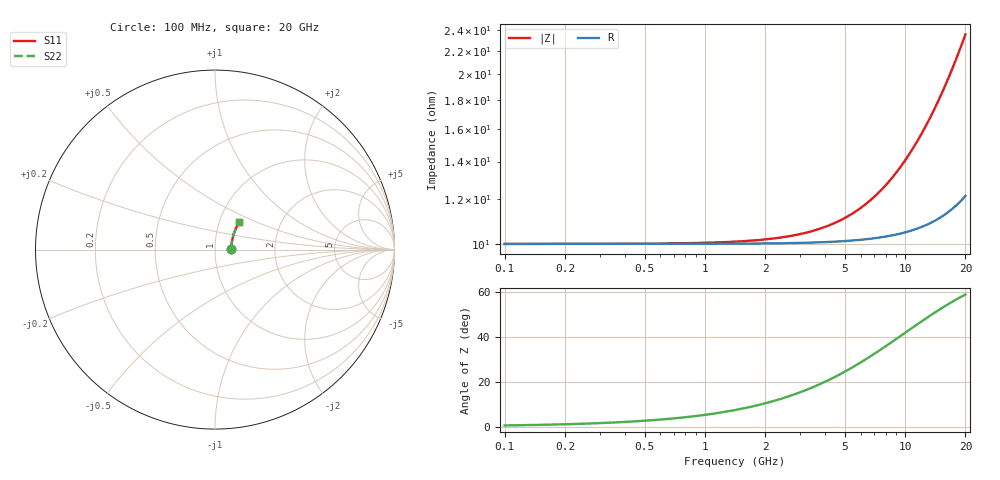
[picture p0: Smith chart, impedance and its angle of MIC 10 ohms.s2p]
! Vishay ElectroFilms Inc.
! MIC001 1000B - 10 Ohm in Series Configuration
! March 2012
# GHz S MA R 50
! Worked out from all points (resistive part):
!   233 points, 100 MHz to 20 GHz, reference 50 ohm
!   read as one part in series: R = 10 ohm at 102.3 MHz
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0.1  0.09091 0.5  0.9091 -0.0  0.9091 -0.0  0.09091 0.5
0.2436751  0.09093 1.2  0.9091 -0.1  0.9091 -0.1  0.09093 1.2
0.5937753  0.09106 2.8  0.9091 -0.3  0.9091 -0.3  0.09106 2.8
1.414214  0.09174 6.7  0.909 -0.7  0.909 -0.7  0.09174 6.7
2.337309  0.09317 11.0  0.9087 -1.1  0.9087 -1.1  0.09317 11.0
2.87065  0.0943 13.4  0.9085 -1.4  0.9085 -1.4  0.0943 13.4
3.446086  0.09576 15.8  0.9083 -1.6  0.9083 -1.6  0.09576 15.8
4.430234  0.09882 19.9  0.9077 -2.1  0.9077 -2.1  0.09882 19.9
4.966127  0.1008 22.0  0.9073 -2.4  0.9073 -2.4  0.1008 22.0
5.566843  0.1032 24.2  0.9069 -2.7  0.9069 -2.7  0.1032 24.2
6.240223  0.1061 26.6  0.9063 -3.0  0.9063 -3.0  0.1061 26.6
6.837118  0.1089 28.5  0.9058 -3.3  0.9058 -3.3  0.1089 28.5
7.664154  0.1132 31.0  0.9049 -3.7  0.9049 -3.7  0.1132 31.0
8.397251  0.1172 33.1  0.904 -4.1  0.904 -4.1  0.1172 33.1
9.413006  0.1232 35.6  0.9027 -4.6  0.9027 -4.6  0.1232 35.6
10.55163  0.1305 38.1  0.901 -5.1  0.901 -5.1  0.1305 38.1
11.82798  0.1392 40.6  0.8989 -5.8  0.8989 -5.8  0.1392 40.6
12.95936  0.1473 42.4  0.8967 -6.4  0.8967 -6.4  0.1473 42.4
14.19896  0.1567 44.1  0.8941 -7.0  0.8941 -7.0  0.1567 44.1
15.9165  0.1705 46.0  0.8899 -7.9  0.8899 -7.9  0.1705 46.0
17.84181  0.1869 47.5  0.8846 -9.0  0.8846 -9.0  0.1869 47.5
20  0.2065 48.7  0.8775 -10.2  0.8775 -10.2  0.2065 48.7
